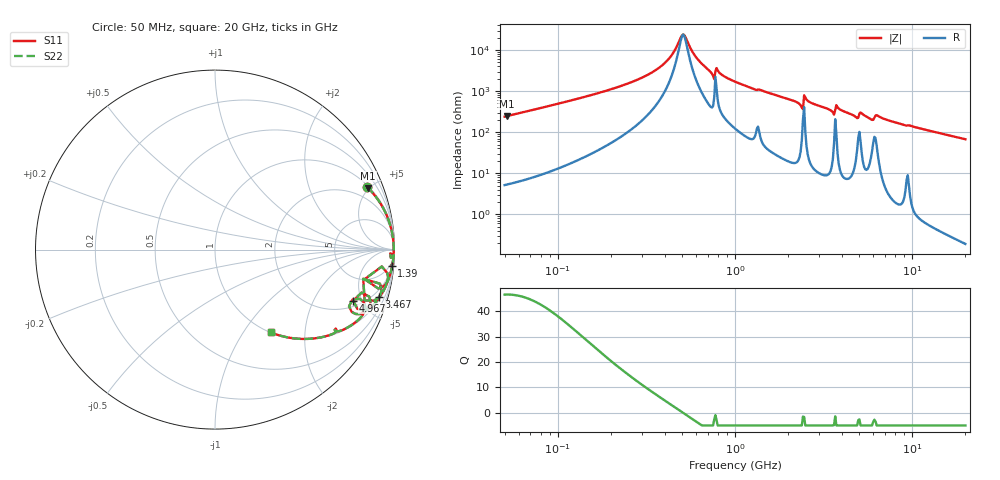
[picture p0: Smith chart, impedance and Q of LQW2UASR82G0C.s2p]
!Murata Part Number: LQW2UASR82G0C
!These Parameters are Measured in Series Mode Connection
!  o--[Z]--o
!Port1  Port2
!  o-------o
!Freq. Start=50[MHz] Stop=20[GHz], 401[Steps]
# Hz S RI R 50
!Freq.(Hz) S11(Real) S11(Imag) S21(Real) S21(Imag) S12(Real) S12(Imag) S22(Real) S22(Imag)
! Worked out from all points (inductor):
!   401 points, 50 MHz to 20 GHz, reference 50 ohm
!   read as one part in series: L = 753 nH near 51.52 MHz
!   highest Q = 46.6 at 51.52 MHz (marker M1), where L = 761 nH
!   self-resonance near 509.6 MHz
!   S11 on the Smith chart (normalised r, x): 50 MHz: 1.10, +4.78; 1.39 GHz: 3, -21; 3.467 GHz: 1.23, -6.82; 4.967 GHz: 2.44, -4.26; 20 GHz: 1.00, -1.34
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5e7  0.8459 0.3505  0.1541 -0.3505  0.1541 -0.3505  0.8459 0.3505
5.152053e7  0.8534 0.3431  0.1466 -0.3431  0.1466 -0.3431  0.8534 0.3431
1.364002e8  0.9752 0.1397  0.0248 -0.1397  0.0248 -0.1397  0.9752 0.1397
2.558771e8  0.992 0.0612  0.00804 -0.0612  0.00804 -0.0612  0.992 0.0612
3.721004e8  0.9951 0.0265  0.00487 -0.0265  0.00487 -0.0265  0.9951 0.0265
4.322267e8  0.9957 0.0138  0.00434 -0.0138  0.00434 -0.0138  0.9957 0.0138
5.096456e8  0.9959 5.94e-05  0.00414 -5.94e-05  0.00414 -5.94e-05  0.9959 5.94e-05
6.009314e8  0.9956 -0.0139  0.00435 0.0139  0.00435 0.0139  0.9956 -0.0139
7.411344e8  0.993 -0.0368  0.007 0.0368  0.007 0.0368  0.993 -0.0368
7.987718e8  0.9932 -0.0305  0.00682 0.0305  0.00682 0.0305  0.9932 -0.0305
1e9  0.9924 -0.0579  0.00758 0.0579  0.00758 0.0579  0.9924 -0.0579
1.390315e9  0.9851 -0.0909  0.0149 0.0909  0.0149 0.0909  0.9851 -0.0909
2.348516e9  0.9393 -0.2039  0.0607 0.2039  0.0607 0.2039  0.9393 -0.2039
2.531158e9  0.9642 -0.1514  0.0358 0.1514  0.0358 0.1514  0.9642 -0.1514
2.728004e9  0.9573 -0.1886  0.0427 0.1886  0.0427 0.1886  0.9573 -0.1886
3.466789e9  0.9134 -0.2651  0.0866 0.2651  0.0866 0.2651  0.9134 -0.2651
3.792786e9  0.9271 -0.2245  0.0729 0.2245  0.0729 0.2245  0.9271 -0.2245
4.966507e9  0.7703 -0.2842  0.2297 0.2842  0.2297 0.2842  0.7703 -0.2842
5.856089e9  0.7829 -0.3585  0.2171 0.3585  0.2171 0.3585  0.7829 -0.3585
6.311513e9  0.8308 -0.2954  0.1692 0.2954  0.1692 0.2954  0.8308 -0.2954
7.442007e9  0.7805 -0.4066  0.2195 0.4066  0.2195 0.4066  0.7805 -0.4066
2e10  0.3116 -0.4618  0.6884 0.4618  0.6884 0.4618  0.3116 -0.4618
